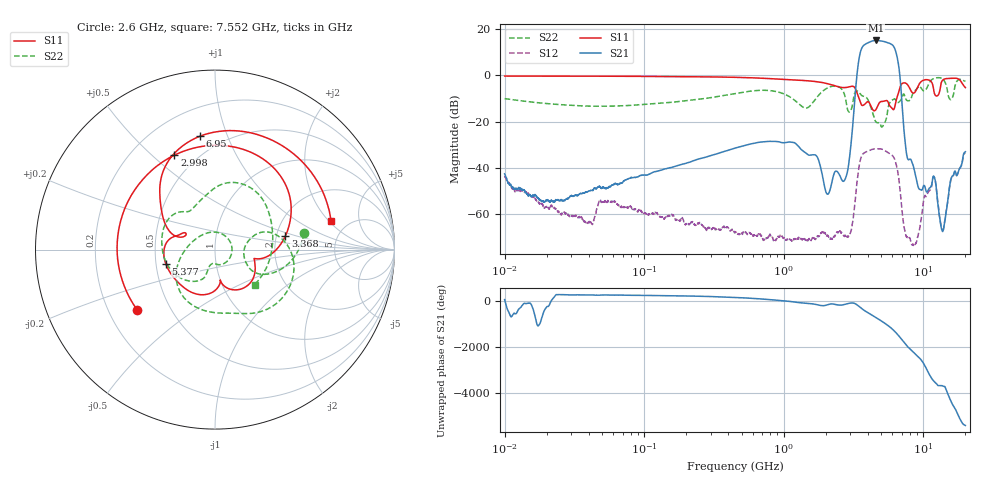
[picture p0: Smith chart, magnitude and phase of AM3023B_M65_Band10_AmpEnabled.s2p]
!Agilent Technologies,E8364B,MY43040894,A.07.50.67
!Agilent E8364B: A.07.50.67
!Date: Tuesday, October 27, 2020 10:54:44
!Correction: S11(Full 2 Port(1,2))
!S21(Full 2 Port(1,2))
!S12(Full 2 Port(1,2))
!S22(Full 2 Port(1,2))
!S2P File: Measurements: S11, S21, S12, S22:Log Frequency Sweep
# Hz S  dB  R 50
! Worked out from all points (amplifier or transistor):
!   3201 points, 10 MHz to 20 GHz, reference 50 ohm
!   highest |S21| = 15.1 dB at 4.554 GHz (marker M1)
!   |S21| within 3 dB of that: 3.642 GHz to 6.182 GHz (2.54 GHz wide, 51.7 % of centre)
!   unconditionally stable (mu >= 1): start of sweep to end of sweep
!   at 35.47 MHz: K = 15224.64, MAG = -39.8 dB, |S12| = -61.1 dB
!   at 447.2 MHz: K = 6821.38, MAG = -23.1 dB, |S12| = -68.0 dB
!   at 20 GHz: K = 333.33, MAG = -28.0 dB, |S12| = -33.5 dB
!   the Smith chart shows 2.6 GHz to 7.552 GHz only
!   S11 on the Smith chart (normalised r, x): 2.6 GHz: 0.32, -0.31; 2.998 GHz: 0.38, +0.59; 3.368 GHz: 2.24, +0.40; 5.377 GHz: 0.56, -0.10; 6.95 GHz: 0.38, +0.80; 7.552 GHz: 3.73, +2.11
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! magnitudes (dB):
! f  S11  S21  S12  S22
! 10 MHz  -0.3  -42.6  -43.9  -10.1
! 18.81 MHz  -0.3  -54.6  -56.5  -12.0
! 35.55 MHz  -0.4  -51.1  -61.3  -13.2
! 126.1 MHz  -0.5  -41.3  -60.4  -12.1
! 447.2 MHz  -0.8  -31.4  -68.0  -7.8
! 1.59 GHz  -2.5  -34.4  -70.7  -12.3
! 2.045 GHz  -3.6  -51.3  -69.3  -5.5
! 2.6 GHz  -5.2  -45.1  -68.0  -5.9
! 2.998 GHz  -4.8  -32.4  -68.1  -15.6
! 3.368 GHz  -8.0  2.0  -44.6  -6.7
! 3.668 GHz  -13.0  12.4  -34.2  -8.9
! 4.554 GHz  -14.9  15.1  -31.7  -20.0
! 5.377 GHz  -10.9  14.4  -32.7  -19.4
! 5.639 GHz  -12.2  14.0  -33.5  -13.0
! 6.411 GHz  -10.4  9.2  -38.8  -11.4
! 6.95 GHz  -3.9  -7.7  -55.6  -10.3
! 7.552 GHz  -3.5  -33.4  -69.6  -10.6
! 8.813 GHz  -6.8  -43.7  -72.6  -6.3
! 11.86 GHz  -6.5  -43.6  -43.7  -1.4
! 13.71 GHz  -2.2  -67.4  -66.6  -1.5
! 15.92 GHz  -1.3  -44.1  -44.1  -10.2
! 20 GHz  -5.3  -33.0  -33.5  -2.6
